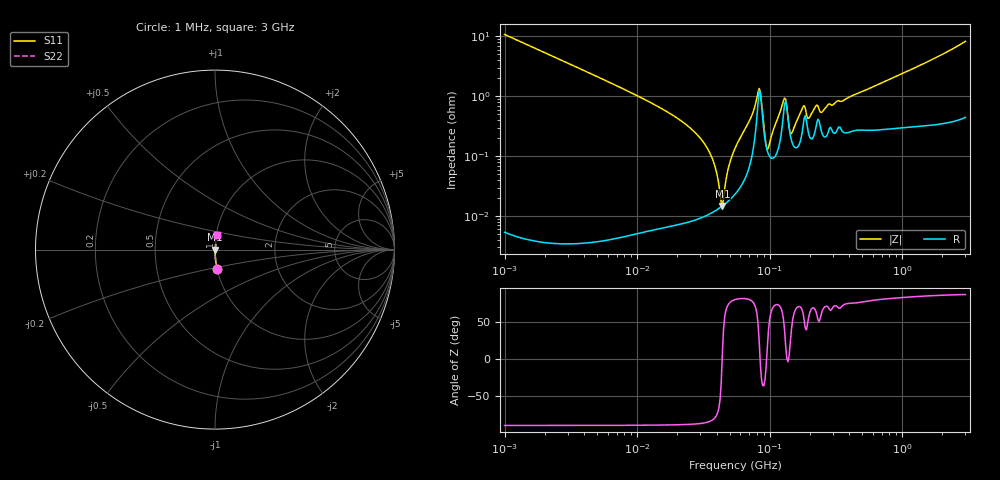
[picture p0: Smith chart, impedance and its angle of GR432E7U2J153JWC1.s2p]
!Murata Part Number: GR432E7U2J153JWC1
!These Parameters are Measured in Series Mode Connection
!Data Generated on Jun 10, 2025
!  o--ll--o
!Port1  Port2
!  o------o
!Operation Temp=25[degC], DC Bias Voltage=0[V]
!Freq. Start=1000[kHz] Stop=3[GHz] 401[Steps]
# Hz S RI R 50
!Freq.(Hz) S11(Real) S11(Imag) S21(Real) S21(Imag) S12(Real) S12(Imag) S22(Real) S22(Imag)
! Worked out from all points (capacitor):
!   401 points, 1 MHz to 3 GHz, reference 50 ohm
!   read as one part in series: C = 14.7 nF near 1.041 MHz
!   lowest |Z| = 14.8 mohm at 43.95 MHz (marker M1)
!   series resonance near 43.83 MHz, so ESL is about 890 pH
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1000000  0.0116 -0.1067  0.9884 0.1067  0.9884 0.1067  0.0116 -0.1067
3823119  0.00082 -0.028  0.9992 0.028  0.9992 0.028  0.00082 -0.028
1.461624e7  0.000105 -0.00661  0.9999 0.00661  0.9999 0.00661  0.000105 -0.00661
3.190472e7  0.000101 -0.00167  0.9999 0.00167  0.9999 0.00167  0.000101 -0.00167
3.74453e7  0.000117 -0.000833  0.9999 0.000833  0.9999 0.000833  0.000117 -0.000833
4.22235e7  0.000138 -0.000201  0.9999 0.000201  0.9999 0.000201  0.000138 -0.000201
4.394807e7  0.000147 1.48e-05  0.9999 -1.48e-05  0.9999 -1.48e-05  0.000147 1.48e-05
4.955604e7  0.000184 0.000696  0.9998 -0.000696  0.9998 -0.000696  0.000184 0.000696
5.477226e7  0.000233 0.00133  0.9998 -0.00133  0.9998 -0.00133  0.000233 0.00133
7.248696e7  0.00089 0.00442  0.9991 -0.00442  0.9991 -0.00442  0.00089 0.00442
8.173662e7  0.00784 0.0085  0.9922 -0.0085  0.9922 -0.0085  0.00784 0.0085
8.507507e7  0.0116 -0.00142  0.9884 0.00142  0.9884 0.00142  0.0116 -0.00142
9.402997e7  0.00149 -0.000297  0.9985 0.000297  0.9985 0.000297  0.00149 -0.000297
9.787052e7  0.00109 0.000842  0.9989 -0.000842  0.9989 -0.000842  0.00109 0.000842
1.269575e8  0.00487 0.00674  0.9951 -0.00674  0.9951 -0.00674  0.00487 0.00674
1.321429e8  0.00841 0.00263  0.9916 -0.00263  0.9916 -0.00263  0.00841 0.00263
1.460522e8  0.00183 0.00151  0.9982 -0.00151  0.9982 -0.00151  0.00183 0.00151
1.784169e8  0.00311 0.00583  0.9969 -0.00583  0.9969 -0.00583  0.00311 0.00583
1.971969e8  0.00235 0.00358  0.9976 -0.00358  0.9976 -0.00358  0.00235 0.00358
2.094008e8  0.00199 0.00498  0.998 -0.00498  0.998 -0.00498  0.00199 0.00498
8.005644e8  0.00319 0.0188  0.9968 -0.0188  0.9968 -0.0188  0.00319 0.0188
3e9  0.0111 0.0815  0.9889 -0.0815  0.9889 -0.0815  0.0111 0.0815
